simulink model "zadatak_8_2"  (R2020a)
settings: Solver=ode23tb  StartTime=0.0  StopTime=0.06  RelTol=1e-3
undefined symbols (not defined in the file): D1, Delta
libraries: powerlib x11

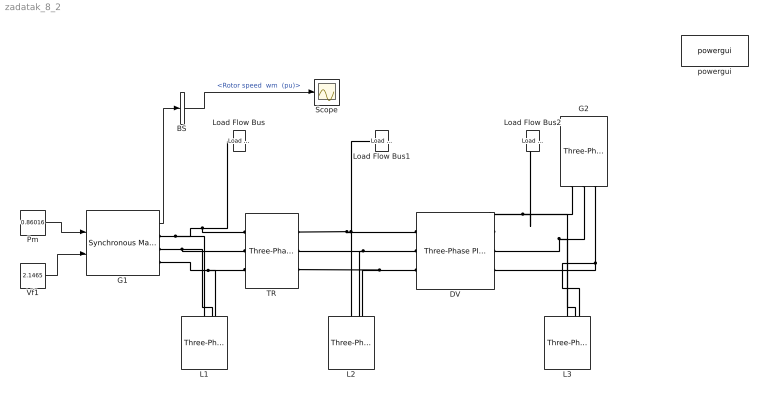
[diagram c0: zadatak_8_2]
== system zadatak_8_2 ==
  BS : BusSelector  OutputSignals="Mechanical.Rotor speed  wm  (pu)"
  DV : powerlib/Elements/Three-Phase PI Section Line  LConnTagsString=a|b|c  RConnTagsString=A|B|C  Frequency=50  Resistances=[ 0.01273 0.3864]  Inductances="[ 0.9337e-3  4.1264e-3]"  Capacitances=[12.74e-9 7.751e-9]  Length=50
  G1 : powerlib/Machines/Synchronous Machine pu Standard  PresetModel=No  MechanicalLoad=Mechanical power Pm  ShowDetailedParameters=on  RotorType=Salient-pole  Units=per unit standard parameters  MeasurementBus=off  NominalParameters=[120e6 15.75e3 50]  Reactances1=[ 1.81, 0.3, 0.23, 1.76, 0.65, 0.25, 0.15 ]  Reactances2=[2.24 0.17 0.12 1.02 0.13 0.08]  dAxisTimeConstants=Short-circuit  qAxisTimeConstants=Short-circuit  TimeConstants1="[ 4.4849  0.0681  0.1  ]"  TimeConstants2=[ 8.0, 0.03, 1.0, 0.07 ]  TimeConstants3="[  4.49  0.0681  0.0513  ]"  TimeConstants4=[ 8.0, 0.03, 0.3371, 0.0295 ]  TimeConstants5=[ 1.01, 0.053, 0.1 ]  TimeConstants6=[ 1.3201, 0.023, 1.0, 0.07 ]  TimeConstants7=[0.012 0.003 0.003]  TimeConstants8=[ 1.3201, 0.0231, 0.3371, 0.0295 ]  StatorResistance=0.037875  Mechanical=[3 0.02056 2]  PolePairs=20  InitialConditions=[0 -77.2497 0.841643 0.841643 0.841643 -31.5874 -151.587 88.4126 2.14653]  SetSaturation=off  Saturation=[0.6404,0.7127,0.8441,0.9214,0.9956,1.082,1.19,1.316,1.457;0.7,0.7698,0.8872,0.9466,0.9969,1.046,1.1,1.151,1.201]  LoadFlowParameters=[1,0,0,0,0]  TsPowergui=0  TsBlock=-1  IterativeModel=Trapezoidal non iterative  IterativeDiscreteModel=Trapezoidal non iterative  BusType=PV  Pref=100e6  Qref=0  Qmin=-inf  Qmax=inf  PLF=0  QLF=0
  G2 : powerlib/Electrical Sources/Three-Phase Source  InternalConnection=Yg  VoltagePhases=off  Voltage=(220000)*1.5706  PhaseAngle=21.1409  Voltage_phases=[25e3 25e3 25e3]/sqrt(3)  PhaseAngles_phases=[0 -120 +120]  Frequency=50  NonIdealSource=on  SpecifyImpedance=on  Resistance=0.8929  Inductance=16.58e-3  ShortCircuitLevel=100e6  BaseVoltage=220e3  XRratio=8  BusType=swing  Pref=10e3  Qref=0  Prefabc=[10e3, 10e3, 10e3]  Qrefabc=[0, 0, 0]  Qmin=-inf  Qmax=inf
  L1 : powerlib/Elements/Three-Phase Series RLC Load  LConnTagsString=A|B|C  Configuration=Y (grounded)  NominalVoltage=15.75e3  Vabc=[1e3 1e3 1e3]  Vabcp=[1e3 1e3 1e3]  NominalFrequency=50  UnbalancedPower=off  ActivePower=5e6  InductivePower=0  CapacitivePower=0  Pabc=[10e3 9e3 11e3]  QLabc=[100 90 110]  QCabc=[100 90 110]  Pabcp=[10e3 9e3 11e3]  QLabcp=[100 90 110]  QCabcp=[100 90 110]  Measurements=None  LoadType=constant Z
  L2 : powerlib/Elements/Three-Phase Series RLC Load  LConnTagsString=A|B|C  Configuration=Y (grounded)  NominalVoltage=220e3  Vabc=[1e3 1e3 1e3]  Vabcp=[1e3 1e3 1e3]  NominalFrequency=50  UnbalancedPower=off  ActivePower=150e6  InductivePower=50e6  CapacitivePower=0  Pabc=[10e3 9e3 11e3]  QLabc=[100 90 110]  QCabc=[100 90 110]  Pabcp=[10e3 9e3 11e3]  QLabcp=[100 90 110]  QCabcp=[100 90 110]  Measurements=None  LoadType=constant Z
  L3 : powerlib/Elements/Three-Phase Series RLC Load  LConnTagsString=A|B|C  Configuration=Y (grounded)  NominalVoltage=220e3  Vabc=[1e3 1e3 1e3]  Vabcp=[1e3 1e3 1e3]  NominalFrequency=50  UnbalancedPower=off  ActivePower=10e6  InductivePower=0  CapacitivePower=0  Pabc=[10e3 9e3 11e3]  QLabc=[100 90 110]  QCabc=[100 90 110]  Pabcp=[10e3 9e3 11e3]  QLabcp=[100 90 110]  QCabcp=[100 90 110]  Measurements=None  LoadType=constant Z
  Load Flow Bus : powerlib/Measurements/Load Flow Bus  LConnTagsString=a  Phases=single  Connectors=on one side  ID=B1  Vbase=15.75e3  Vref=1  Vangle=0  VLF=1  VLFb=1  VLFc=1  angleLF=-23.53  angleLFb=0  angleLFc=0
  Load Flow Bus1 : powerlib/Measurements/Load Flow Bus  LConnTagsString=a  Phases=single  Connectors=on one side  ID=B2  Vbase=220e3  Vref=1  Vangle=0  VLF=0.9862  VLFb=1  VLFc=1  angleLF=-0.8729  angleLFb=0  angleLFc=0
  Load Flow Bus2 : powerlib/Measurements/Load Flow Bus  LConnTagsString=a  Phases=single  Connectors=on one side  ID=B3  Vbase=220e3  Vref=1  Vangle=0  VLF=1  VLFb=1  VLFc=1  angleLF=0  angleLFb=0  angleLFc=0
  Pm : Constant  Value=0.86016
  Scope : Scope
  TR : powerlib/Elements/Three-Phase Transformer (Two Windings)  Winding1Connection=Delta (D1)  Winding2Connection=Yg  CoreType=Three-limb core (core-type)  SetSaturation=off  Hysteresis=off  DataFile='hysteresis'  SetInitialFlux=off  Measurements=None  UNITS=pu  NominalPower=[ 120e6 , 50 ]  Winding1=[ 15.75e3 , 0.002 , 0.08 ]  Winding2=[ 220e3 , 0.002 , 0.08 ]  Rm=500  Lm=500  L0=0.5  Saturation=[ 0,0 ; 0.0024,1.2 ; 1.0,1.52 ]  InitialFluxes=[ 0.8 , -0.8 , 0.7 ]  BreakLoop=off  DiscreteSolver=Trapezoidal iterative  DataType=off  TransfoNumber=1
  Vf1 : Constant  Value=2.1465
  powergui : powerlib/powergui  Priority=1  SimulationMode=Continuous  SampleTime=50e-6  frequency=60  Iterations=50  frequencyindice=50  Pbase=100e6  ErrMax=1e-06  UnitsV=kV  UnitsW=MW  buscounter=0  FunctionMessages=off  echomessages=off  EnableUseOfTLC=off  CurrentSourceSwitches=off  DisableSnubberDevices=off  DisableRonSwitches=off  DisableVfSwitches=off  DisplayEquations=off  AutomaticDiscreteSolvers=off  SolverType=Tustin/Backward Euler (TBE)  Interpol=off  ExternalGateDelay=off  methode=off  Ts=100  x0status=blocks  SPID=on  SwTol=0  HookPort=off  NonlinearTolerance=1e-4  nMaxIteration=100  ContinueOnMaxIteration=off  RestoreLinks=warning  ResistiveCurrentMeasurement=off  Frange=[0:2:500]  Ylog=off  Xlog=on  ShowGrid=off  save=off  variable=ZData  structure=0  ZoomFFT=off  StartTime=0.0  cycles=1  DisplayStyle=1  fundamental=60  FreqAxis=off  MaxFrequency=1000  frequencyindicesteady=1  RmsSteady=1  display=off
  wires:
  Pm/1 -> G1/1
  Vf1/1 -> G1/2
  G1/1 -> BS/1
  BS/1 -> Scope/1  "<Rotor speed  wm  (pu)>"
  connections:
  G1/RConn1 -- L1/LConn1 -- Load Flow Bus/LConn1 -- TR/LConn1
  G1/RConn2 -- TR/LConn2 -- L1/LConn2
  G1/RConn3 -- L1/LConn3 -- TR/LConn3
  DV/LConn1 -- Load Flow Bus1/LConn1 -- TR/RConn1 -- L2/LConn1
  DV/LConn2 -- TR/RConn2 -- L2/LConn2
  DV/LConn3 -- TR/RConn3 -- L2/LConn3
  G2/RConn1 -- L3/LConn1 -- Load Flow Bus2/LConn1 -- DV/RConn1
  G2/RConn2 -- DV/RConn2 -- L3/LConn2
  G2/RConn3 -- L3/LConn3 -- DV/RConn3
